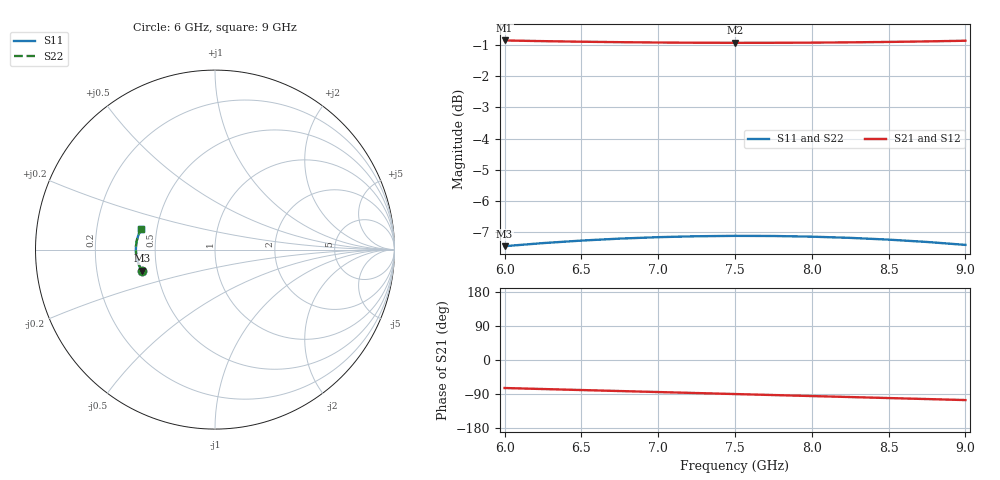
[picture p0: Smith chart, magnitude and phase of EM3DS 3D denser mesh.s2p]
!AWR Design Environment (2469) Mon Oct 04 18:05:22 2004
!freq-unit  param-type  data-format  keyword  impedance-ohms
# GHz  S  MA  R  50
!Freq  MagS11  AngS11  MagS21  AngS21  MagS12  AngS12  MagS22  AngS22
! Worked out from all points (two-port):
!   13 points, 6 GHz to 9 GHz, reference 50 ohm
!   highest |S21| = -0.86 dB at 6 GHz (marker M1); lowest = -0.9 dB at 7.5 GHz (marker M2)
!   |S21| within 3 dB of the highest: start of sweep to end of sweep
!   lowest |S11| = -7.4 dB at 6 GHz (marker M3), VSWR 2.47, Z = 20.5 - j5.88 ohm
!   |S11| at or under -10 dB: nowhere
!   |S22| runs from -7.4 to -7.1 dB; largest |S21 - S12| = 0
6  0.4244 -163.9  0.9055 -73.9  0.9055 -73.9  0.4244 -163.9
6.25  0.4292 -166.6  0.9032 -76.6  0.9032 -76.6  0.4292 -166.6
6.5  0.4332 -169.3  0.9013 -79.3  0.9013 -79.3  0.4332 -169.3
6.75  0.4364 -171.9  0.8998 -81.9  0.8998 -81.9  0.4364 -171.9
7  0.4387 -174.6  0.8986 -84.6  0.8986 -84.6  0.4387 -174.6
7.25  0.4402 -177.2  0.8979 -87.2  0.8979 -87.2  0.4402 -177.2
7.5  0.4408 -179.8  0.8976 -89.8  0.8976 -89.8  0.4408 -179.8
7.75  0.4406 177.5  0.8977 -92.5  0.8977 -92.5  0.4406 177.5
8  0.4395 174.9  0.8982 -95.1  0.8982 -95.1  0.4395 174.9
8.25  0.4376 172.2  0.8992 -97.8  0.8992 -97.8  0.4376 172.2
8.5  0.4347 169.6  0.9006 -100.4  0.9006 -100.4  0.4347 169.6
8.75  0.431 166.9  0.9023 -103.1  0.9023 -103.1  0.431 166.9
9  0.4264 164.3  0.9045 -105.7  0.9045 -105.7  0.4264 164.3
